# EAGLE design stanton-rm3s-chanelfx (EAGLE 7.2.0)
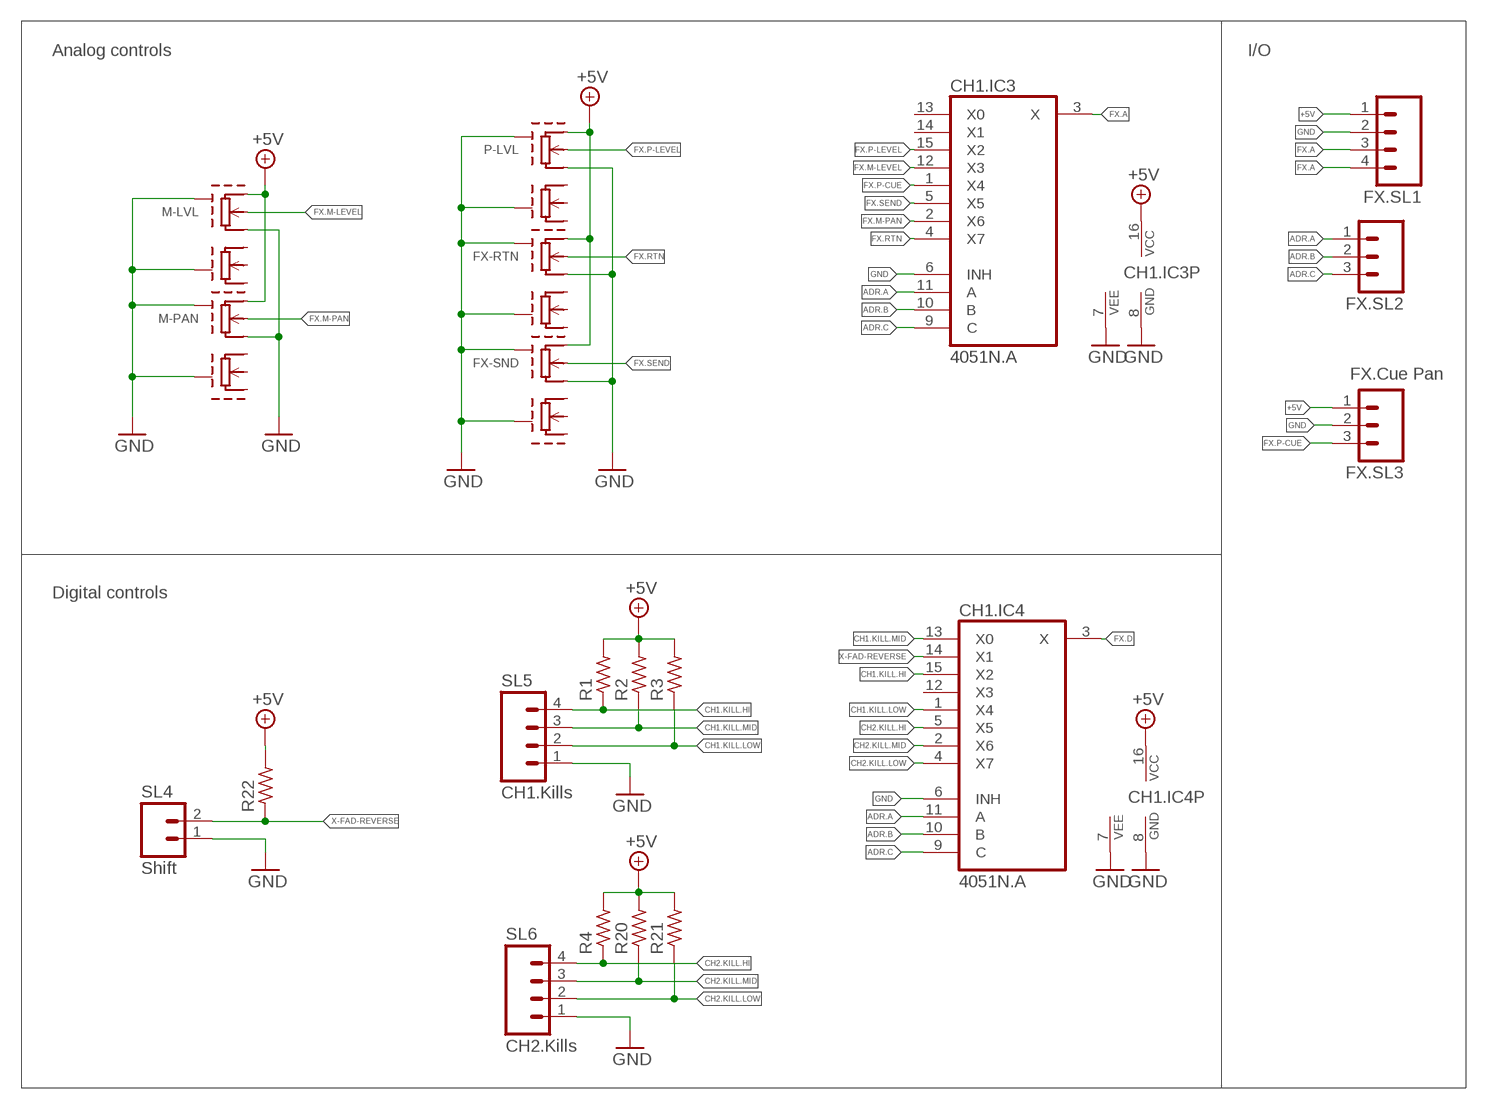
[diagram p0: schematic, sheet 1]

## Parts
CH1.IC3  4051N.A  4051N  [DIL16]
CH1.IC4  4051N.A  4051N  [DIL16]
FX-RTN  RM3S-POTRM3S-POT  [RM3S-POT]
FX-SND  RM3S-POTRM3S-POT  [RM3S-POT]
FX.SL1  M04  [04P]
FX.SL2  M03  [03P]
FX.SL3  FX.Cue Pan  M03  [03P]
M-LVL  RM3S-POTRM3S-POT  [RM3S-POT]
M-PAN  RM3S-POTRM3S-POT  [RM3S-POT]
P-LVL  RM3S-POTRM3S-POT  [RM3S-POT]
R1  R-EU_0207/10C  [0207/10C]
R2  R-EU_0207/10C  [0207/10C]
R3  R-EU_0207/10C  [0207/10C]
R4  R-EU_0207/10C  [0207/10C]
R20  R-EU_0207/10C  [0207/10C]
R21  R-EU_0207/10C  [0207/10C]
R22  R-EU_0207/10C  [0207/10C]
SL4  Shift  M02  [02P]
SL5  CH1.Kills  M04  [04P]
SL6  CH2.Kills  M04  [04P]

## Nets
+5V: CH1.IC3.16(VCC) CH1.IC4.16(VCC) FX-RTN.1 FX-SND.1 FX.SL1.1 FX.SL3.1 M-LVL.1 M-PAN.1 P-LVL.1 R1.2 R2.2 R3.2 R4.2 R20.2 R21.2 R22.2
ADR.A: CH1.IC3.11(A) CH1.IC4.11(A) FX.SL2.1
ADR.B: CH1.IC3.10(B) CH1.IC4.10(B) FX.SL2.2
ADR.C: CH1.IC3.9(C) CH1.IC4.9(C) FX.SL2.3
CH1.KILL.HI: CH1.IC4.15(X2) R1.1 SL5.4
CH1.KILL.LOW: CH1.IC4.1(X4) R3.1 SL5.2
CH1.KILL.MID: CH1.IC4.13(X0) R2.1 SL5.3
CH2.KILL.HI: CH1.IC4.5(X5) R4.1 SL6.4
CH2.KILL.LOW: CH1.IC4.4(X7) R21.1 SL6.2
CH2.KILL.MID: CH1.IC4.2(X6) R20.1 SL6.3
FX.A: CH1.IC3.3(X) FX.SL1.3
FX.D: CH1.IC4.3(X) FX.SL1.4
FX.M-LEVEL: CH1.IC3.12(X3) M-LVL.6
FX.M-PAN: CH1.IC3.2(X6) M-PAN.6
FX.P-CUE: CH1.IC3.1(X4) FX.SL3.3
FX.P-LEVEL: CH1.IC3.15(X2) P-LVL.6
FX.RTN: CH1.IC3.4(X7) FX-RTN.6
FX.SEND: CH1.IC3.5(X5) FX-SND.6
GND: CH1.IC3.6(INH) CH1.IC3.7(VEE) CH1.IC3.8(GND) CH1.IC4.6(INH) CH1.IC4.7(VEE) CH1.IC4.8(GND) FX-RTN.5 FX-RTN.GND1 FX-RTN.GND2 FX-SND.5 FX-SND.GND1 FX-SND.GND2 FX.SL1.2 FX.SL3.2 M-LVL.5 M-LVL.GND1 M-LVL.GND2 M-PAN.5 M-PAN.GND1 M-PAN.GND2 P-LVL.5 P-LVL.GND1 P-LVL.GND2 SL4.1 SL5.1 SL6.1
X-FAD-REVERSE: CH1.IC4.14(X1) R22.1 SL4.2
Unconnected: CH1.IC3.13(X0) CH1.IC3.14(X1) CH1.IC4.12(X3) FX-RTN.2 FX-RTN.3 FX-RTN.4 FX-SND.2 FX-SND.3 FX-SND.4 M-LVL.2 M-LVL.3 M-LVL.4 M-PAN.2 M-PAN.3 M-PAN.4 P-LVL.2 P-LVL.3 P-LVL.4

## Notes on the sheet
- Analog controls | I/O
- Digital controls

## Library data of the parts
CH1.IC3 CH1.IC4 = 40xx:4051: 8-channel ANALOG MULTIPLEXER
FX-RTN FX-SND M-LVL M-PAN P-LVL = stanton-rm3s:RM3S-POT
FX.SL1 SL5 SL6 = con-amp-quick:M04: AMP QUICK CONNECTOR
FX.SL2 FX.SL3 = con-amp-quick:M03: AMP QUICK CONNECTOR
R1-R4 R20-R22 = rcl:R-EU_: RESISTOR, European symbol
SL4 = con-amp-quick:M02: AMP QUICK CONNECTOR

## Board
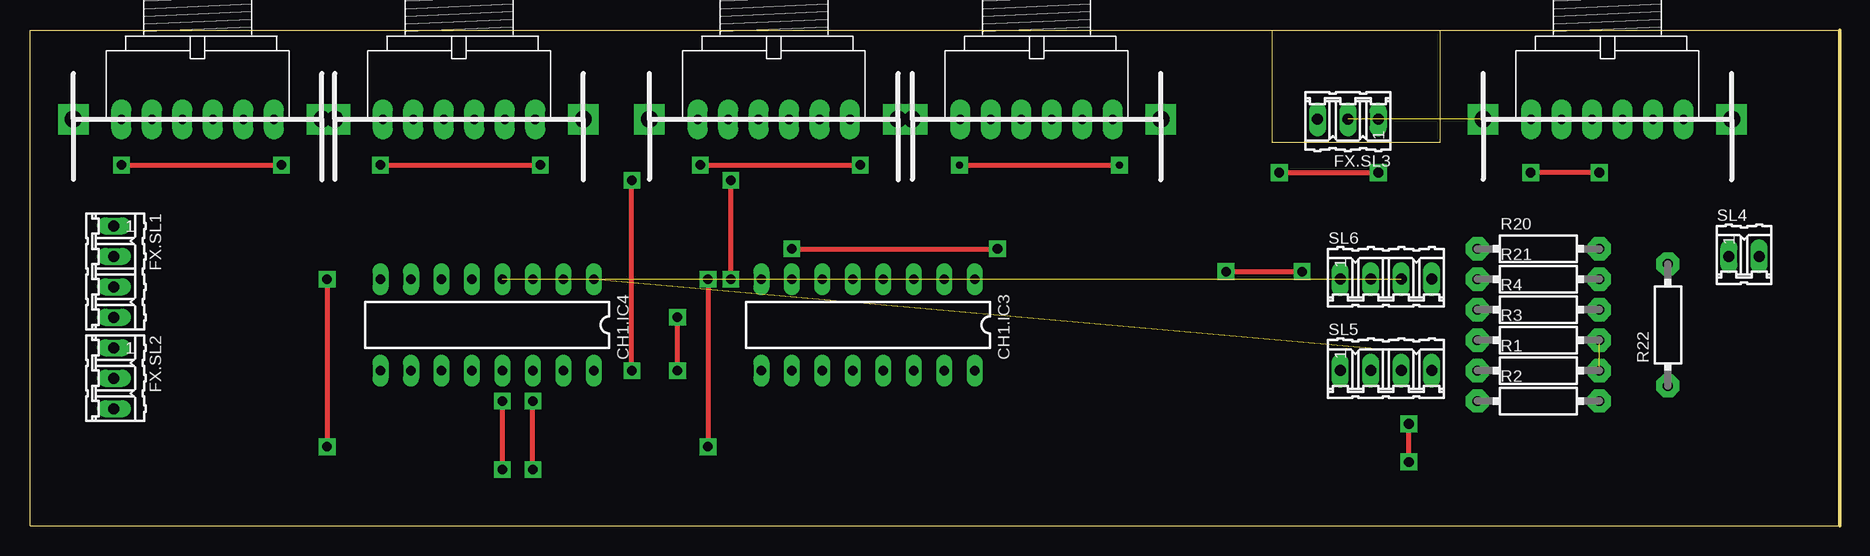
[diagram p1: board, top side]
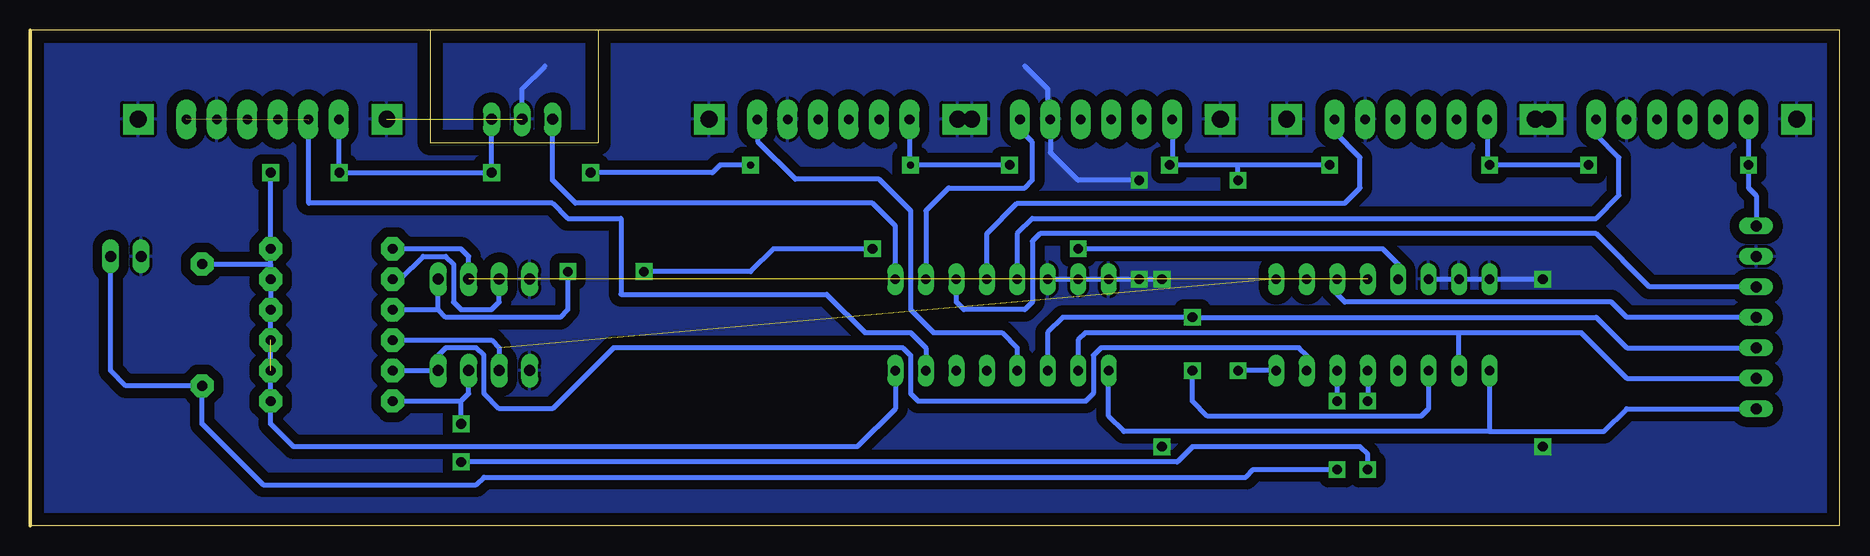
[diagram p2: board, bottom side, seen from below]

Size 150.87 x 41.35 mm. Coordinates in mm from the lower left corner, seen from the top.
Outline: 103.51,41.35 0,41.35 0,0 150.87,0 150.87,41.35 117.53,41.35
Outline: 103.51,41.35 117.53,41.35
Outline: 103.53,31.94 117.53,31.94 117.53,41.35
Outline: 103.51,41.35 103.51,31.94
Copper layers (1*16): Top 0.035mm / dielectric 1.5mm / Bottom 0.035mm
Design rules "default": minimum track width 10mil, minimum drill 24mil, track to track 8mil, track to pad 8mil, pad to pad 8mil, via to via 8mil, smd to smd 8mil, copper to edge 40mil, drill to drill 8mil, minimum pad ring 10mil, minimum via ring 8mil, stop-mask expansion 4mil, vias tented up to drill 0mil, thermal gap 10mil

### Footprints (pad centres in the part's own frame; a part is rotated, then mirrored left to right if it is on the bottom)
DIL16 = drill 0.813 long: 1 -8.89,-3.81; 2 -6.35,-3.81; 3 -3.81,-3.81; 4 -1.27,-3.81; 5 1.27,-3.81; 6 3.81,-3.81; 7 6.35,-3.81; 8 8.89,-3.81; 9 8.89,3.81; 10 6.35,3.81; 11 3.81,3.81; 12 1.27,3.81; 13 -1.27,3.81; 14 -3.81,3.81; 15 -6.35,3.81; 16 -8.89,3.81
RM3S-POT = drill 0.8 pad 1.676 long: 1 -6.35,0; 2 -3.81,0; 3 -1.27,0; 4 1.27,0; 5 3.81,0; 6 6.35,0 | drill 1.4 pad 2.54 square: GND1 -10.36,0; GND2 10.36,0
04P = drill 0.914 long: 1 -3.81,0; 2 -1.27,0; 3 1.27,0; 4 3.81,0
03P = drill 0.914 long: 1 -2.54,0; 2 0,0; 3 2.54,0
0207/10C = drill 0.813 pad 1.93 octagon: 1 -5.08,0; 2 5.08,0
02P = drill 0.914 long: 1 -1.27,0; 2 1.27,0

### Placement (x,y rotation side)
CH1.IC3  69.85,16.75 180 top
CH1.IC4  38.1,16.75 180 top
FX-RTN  35.76,33.91 0 top
FX-SND  13.97,33.91 0 top
FX.SL1  6.99,21.2 270 top
FX.SL2  6.99,12.31 270 top
FX.SL3  109.85,33.9 180 top
M-LVL  83.9,33.91 0 top
M-PAN  62,33.91 0 top
P-LVL  131.49,33.91 0 top
R1  125.73,12.94 0 top
R2  125.73,10.4 0 top
R3  125.73,15.48 0 top
R4  125.73,18.02 0 top
R20  125.73,23.1 0 top
R21  125.73,20.56 0 top
R22  136.53,16.75 90 top
SL4  142.88,22.47 0 top
SL5  113.03,12.94 0 top
SL6  113.03,20.56 0 top

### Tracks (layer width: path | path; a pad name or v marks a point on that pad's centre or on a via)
+5V  (via drill 0.6 pad 1.4, 0.8 pad 1.4)  (1 unrouted)
  Top 0.406: v7.62,30.09 v20.96,30.09 | v29.21,30.09 v42.55,30.09 | v55.88,30.09 v69.21,30.09 | v77.47,30.09 v90.81,30.09 | v130.81,29.45 v125.09,29.45 | v50.17,12.94 v50.17,28.81 | v104.14,29.45 v112.4,29.45
  Bottom 0.406: v20.96,30.09 v29.21,30.09 | v42.55,30.09 50.17,30.09 | 50.17,30.09 v55.88,30.09 | v69.21,30.09 v77.47,30.09 | v90.81,30.09 93.34,30.09 93.98,29.45 v104.14,29.45 | 55.66,30.31 v55.88,30.09 | 29.42,30.29 v29.21,30.09 | 77.55,30.17 v77.47,30.09 | R21.2 R20.2 v130.81,29.45 | R22.2 130.81,21.83 R21.2 | R21.2 R4.2 R1.2 R2.2 130.81,8.5 128.91,6.59 81.92,6.59 78.74,9.77 CH1.IC3.16 | CH1.IC4.16 v50.17,12.94 | v50.17,28.81 50.17,30.09 | FX.SL1.1 6.99,27.55 7.62,28.18 v7.62,30.09 FX-SND.1 | FX-RTN.1 29.41,30.28 v29.21,30.09 | M-PAN.1 55.65,30.31 v55.88,30.09 | M-LVL.1 77.55,30.17 v77.47,30.09 | P-LVL.1 125.14,29.49 v125.09,29.45 v112.4,29.45 FX.SL3.1
ADR.A  (via drill 0.8 pad 1.4)
  Top 0.406: v53.97,12.94 v53.97,17.39
  Bottom 0.406: CH1.IC3.11 66.04,16.12 64.77,17.39 v53.97,17.39 20.32,17.39 17.78,14.85 FX.SL2.1 | CH1.IC4.11 34.29,9.77 34.93,9.13 52.7,9.13 53.97,10.4 v53.97,12.94
ADR.B
  Bottom 0.406: CH1.IC3.10 63.5,15.48 62.87,16.12 31.75,16.12 | 31.75,16.12 21.59,16.12 17.78,12.31 FX.SL2.2 | CH1.IC4.10 31.75,16.12
ADR.C
  Bottom 0.406: CH1.IC4.9 29.21,7.86 | 29.21,7.86 59.69,7.86 60.96,9.13 CH1.IC3.9 | 29.21,7.86 19.69,7.86 17.78,9.77 FX.SL2.3
CH1.KILL.HI
  Bottom 0.406: CH1.IC4.15 44.45,14.21 45.09,14.85 61.59,14.85 62.23,14.21 62.23,11.04 62.87,10.4 76.83,10.4 77.47,11.04 77.47,14.21 78.1,14.85 102.24,14.85 107.31,9.77 111.76,9.77 113.03,11.04 113.03,14.21 113.67,14.85 116.2,14.85 116.84,14.21 SL5.4 R1.1
CH1.KILL.LOW  (1 unrouted)
  Bottom 0.406: R3.1 112.4,15.48 111.76,14.85 SL5.2
CH1.KILL.MID  (via drill 0.8 pad 1.4)
  Top 0.406: v39.37,10.4 v39.37,4.69 | v114.94,5.32 v114.94,8.5
  Bottom 0.406: R2.1 114.94,10.4 | 114.94,10.4 114.3,11.04 SL5.3 | CH1.IC4.13 v39.37,10.4 | v39.37,4.69 39.37,5.96 40,6.59 53.97,6.59 55.25,5.32 v114.94,5.32 | v114.94,8.5 114.94,10.4
CH2.KILL.HI  (via drill 0.8 pad 1.4)
  Top 0.406: v63.5,23.1 v80.65,23.1 | v99.69,21.2 v106.05,21.2
  Bottom 0.406: CH1.IC4.5 36.83,21.83 38.1,23.1 v63.5,23.1 | v80.65,23.1 88.9,23.1 90.81,21.2 v99.69,21.2 | v106.05,21.2 106.05,18.02 106.68,17.39 116.2,17.39 116.84,18.02 | 116.84,18.02 SL6.4 | R4.1 116.84,18.02
CH2.KILL.LOW  (1 unrouted)
  Bottom 0.406: R21.1 120.02,20.56 118.11,22.47 116.2,22.47 115.57,21.83 115.57,18.66 114.94,18.02 112.4,18.02 111.76,18.66 SL6.2
CH2.KILL.MID  (1 unrouted)
  Bottom 0.406: SL6.3 114.3,22.47 114.94,23.1 R20.1
FX.A
  Bottom 0.406: FX.SL1.3 15.88,19.93 20.32,24.37 66.68,24.37 67.31,23.74 67.31,18.66 67.94,18.02 73.03,18.02 73.66,18.66 CH1.IC3.3
FX.D
  Bottom 0.406: FX.SL1.4 17.78,17.39 19.05,18.66 41.28,18.66 41.91,19.29 CH1.IC4.3
FX.M-LEVEL
  Bottom 0.406: CH1.IC3.12 68.58,14.85 69.85,16.12 75.56,16.12 77.47,18.02 77.47,26.28 80.09,28.9 87.07,28.9 90.17,31.99 90.17,33.82 M-LVL.6
FX.M-PAN
  Bottom 0.406: CH1.IC3.2 76.2,26.28 74.3,28.18 67.94,28.18 67.31,28.81 67.31,31.99 68.35,33.03 M-PAN.6
FX.P-CUE
  Bottom 0.406: CH1.IC3.1 78.74,25 80.65,26.91 105.41,26.91 107.31,28.81 FX.SL3.3
FX.P-LEVEL  (1 unrouted)
  Bottom 0.406: CH1.IC3.15 76.2,14.85 77.47,16.12 81.28,16.12 84.45,19.29 101.6,19.29 101.6,25.64 106.05,25.64 107.31,26.91 127.64,26.91 127.64,33.85
FX.RTN
  Bottom 0.406: CH1.IC3.4 71.12,24.37 68.58,26.91 41.28,26.91 40,28.18 40,30.72 42.11,32.82 FX-RTN.6
FX.SEND
  Bottom 0.406: CH1.IC3.5 68.58,24.37 67.31,25.64 20.32,25.64 18.42,27.55 18.42,30.72 20.32,32.62 FX-SND.6
GND  (via drill 0.8 pad 1.4)  (1 unrouted)
  Top 0.406: v56.52,20.56 v56.52,6.59 | v24.77,20.56 v24.77,6.59 | v58.42,20.56 v58.42,28.81
  Bottom 0.406: v56.52,20.56 v58.42,20.56 CH1.IC3.8 CH1.IC3.6 | CH1.IC4.6 v24.77,20.56 | v58.42,28.81 63.5,28.81 65.81,31.13 65.81,33.26 | M-PAN.5 65.81,33.26 | FX.SL3.2 109.85,36.44 107.95,38.34 | 67.94,38.34 66.04,36.44 66.04,33.49 65.81,33.26
  pour Bottom (isolate 0.813): 0.63,40.88 0.63,0.24 150.5,0.24 150.5,40.88
X-FAD-REVERSE  (via drill 0.8 pad 1.4)
  Top 0.406: v41.91,4.69 v41.91,10.4
  Bottom 0.406: SL4.2 144.15,12.94 142.88,11.67 R22.1 136.53,8.5 131.44,3.42 113.67,3.42 113.03,4.05 49.53,4.05 48.9,4.69 v41.91,4.69 | v41.91,10.4 CH1.IC4.14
